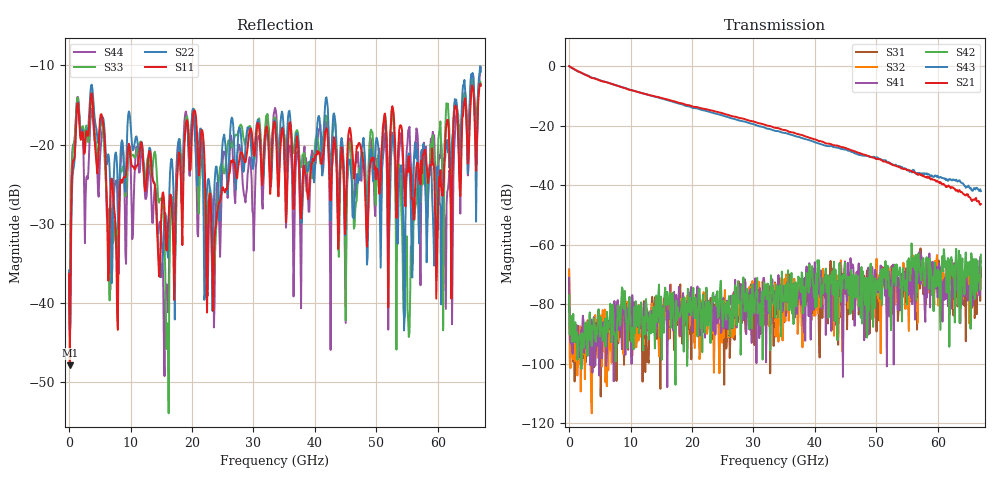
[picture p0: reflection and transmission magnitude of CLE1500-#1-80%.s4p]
!Keysight Technologies,N5247B,US50470101,A.16.20.02
!Date: Thursday, March 13, 2025 10:30:07
!Correction: S11(C  4-Port  )
!S12(C  4-Port  )
!S13(C  4-Port  )
!S14(C  4-Port  )
!S21(C  4-Port  )
!S22(C  4-Port  )
!S23(C  4-Port  )
!S24(C  4-Port  )
!S31(C  4-Port  )
!S32(C  4-Port  )
!S33(C  4-Port  )
!S34(C  4-Port  )
!S41(C  4-Port  )
!S42(C  4-Port  )
!S43(C  4-Port  )
!S44(C  4-Port  )
!S4P File: Measurements: <S11,S12,S13,S14>,
!<S21,S22,S23,S24>,
!<S31,S32,S33,S34>,
!<S41,S42,S43,S44>:
# Hz S  dB  R 50
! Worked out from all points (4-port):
!   601 points, 10 MHz to 67 GHz, reference 50 ohm
!   strongest paths, dB at 10 MHz, 16.76 GHz, 33.51 GHz, 50.25 GHz, 67 GHz:
!     S21: 0.0, -11.6, -20.7, -31.2, -46.3
!     S43: 0.0, -11.9, -21.7, -30.8, -42.0
!     S42: -77.0, -76.7, -84.4, -74.8, -63.3
!     S41: -71.1, -85.3, -75.6, -76.0, -65.9
!     S32: -68.6, -78.7, -73.0, -78.0, -68.9
!     S31: -68.3, -76.8, -72.6, -76.5, -67.6
!   lowest |S11| = -47.9 dB at 121.7 MHz (marker M1), VSWR 1.01, Z = 50.4 - j0.0284 ohm
!   |S11| at or under -10 dB: start of sweep to end of sweep
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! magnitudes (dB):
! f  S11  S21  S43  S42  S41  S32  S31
! 10 MHz  -36.3  0.0  0.0  -77.0  -71.1  -68.6  -68.3
! 121.7 MHz  -47.9  -0.1  -0.2  -90.2  -90.9  -99.2  -88.2
! 3.694 GHz  -13.5  -4.0  -3.8  -94.0  -92.4  -116.6  -92.1
! 15.98 GHz  -32.0  -11.2  -11.4  -75.8  -107.9  -83.4  -92.3
! 52.6 GHz  -15.2  -33.2  -33.0  -73.0  -67.2  -72.9  -83.1
! 55.39 GHz  -23.5  -35.0  -35.5  -68.1  -67.1  -69.6  -79.3
! 67 GHz  -12.6  -46.3  -42.0  -63.3  -65.9  -68.9  -67.6
